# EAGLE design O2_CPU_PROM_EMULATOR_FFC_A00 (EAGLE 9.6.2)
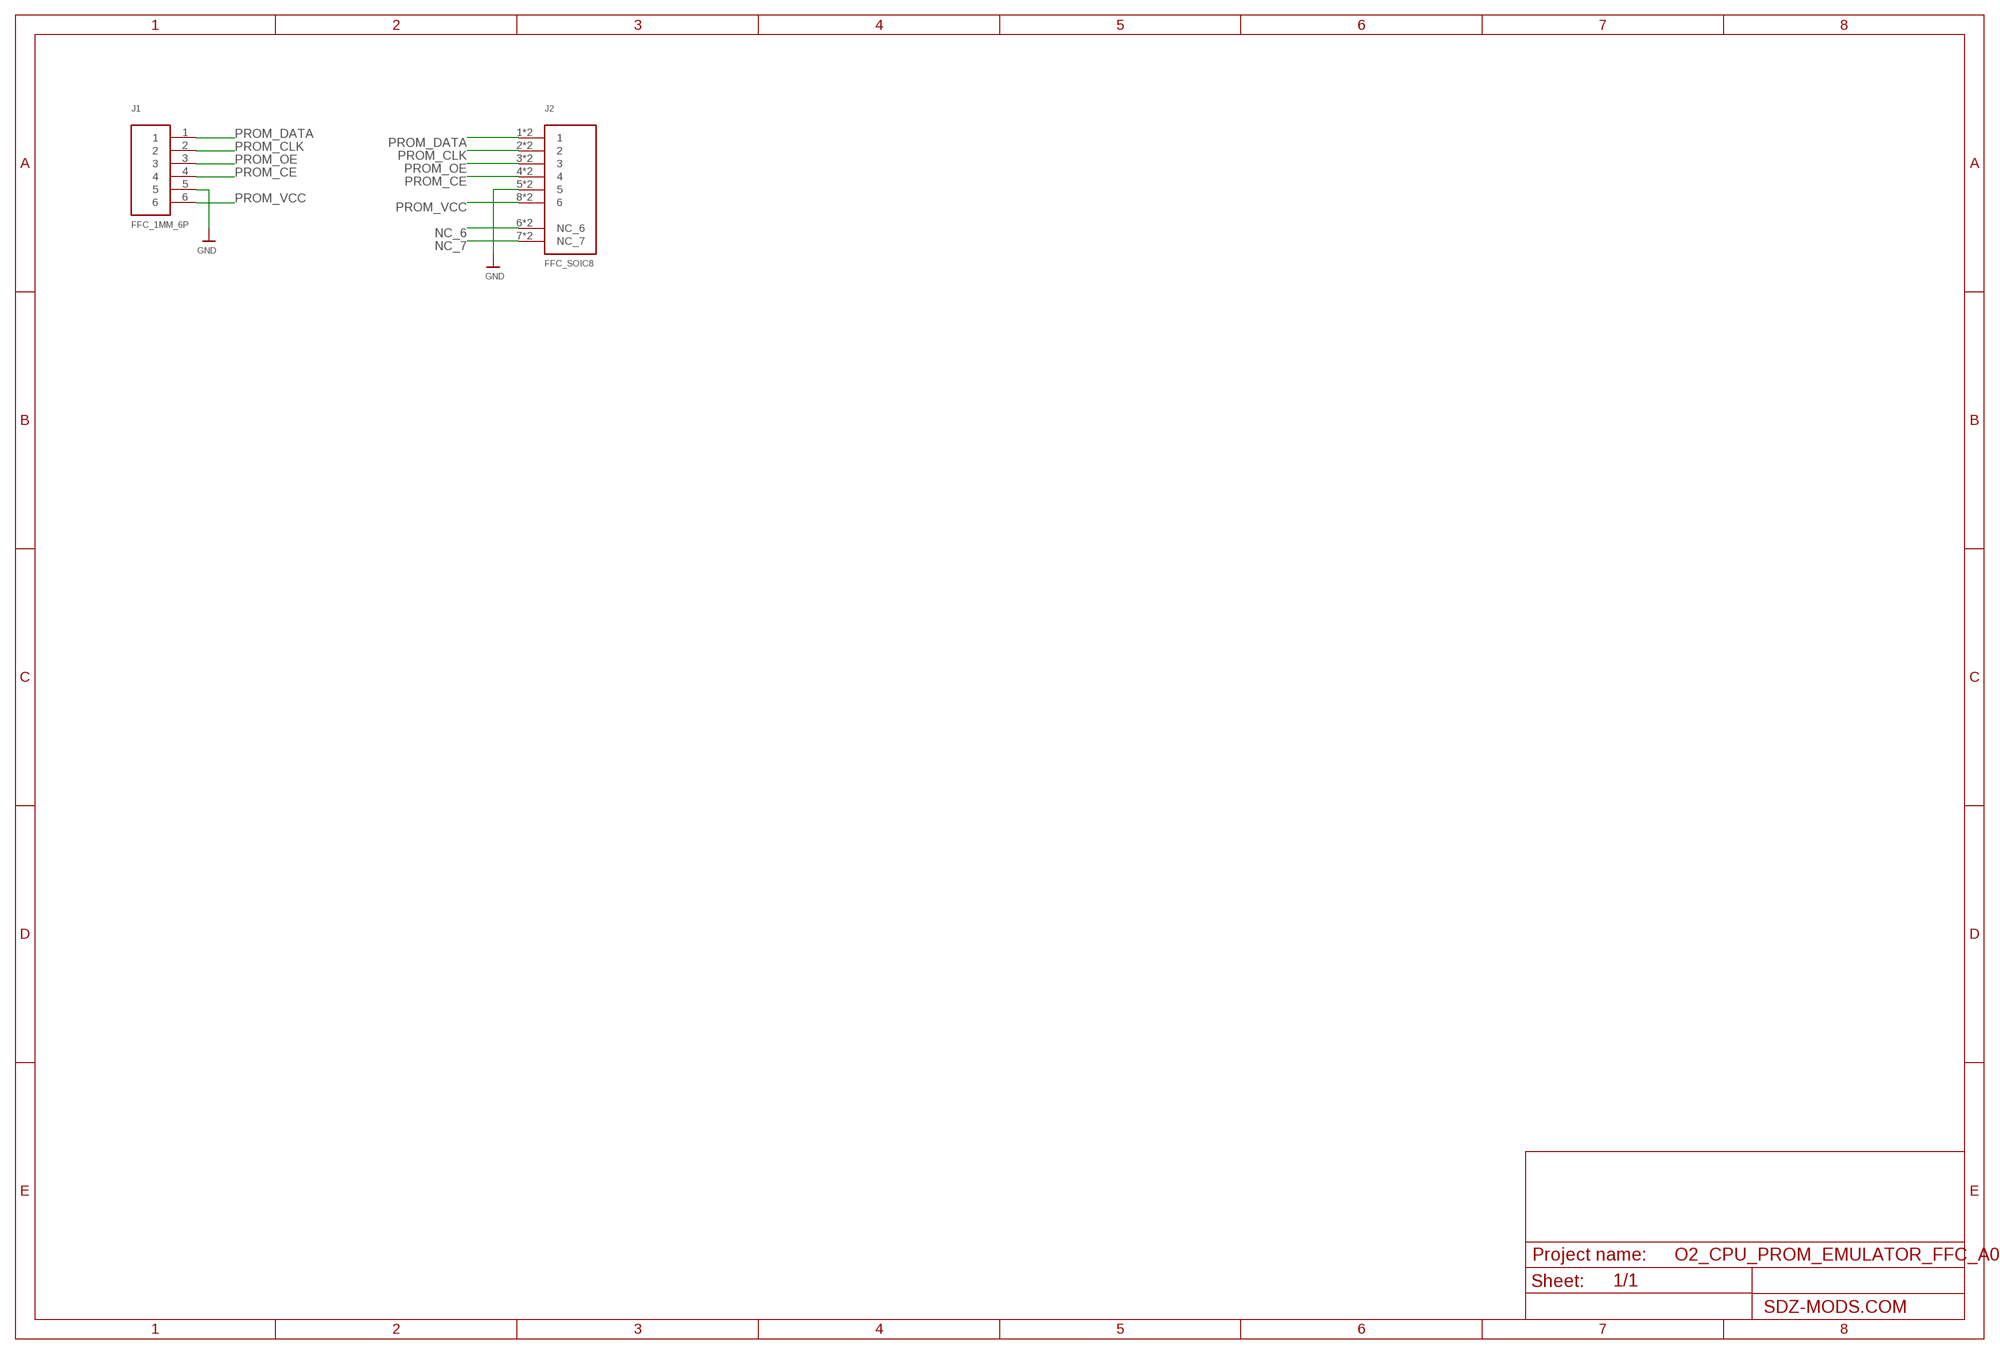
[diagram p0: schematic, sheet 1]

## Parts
J1  FFC_1MM_6P  [FFC_1MM_6P]
J2  FFC_SOIC8  [FFC_SOIC8]

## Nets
GND: J1.5 J2.5 J2.5B
NC_6: J2.6(NC_6) J2.6B(NC_6)
NC_7: J2.7(NC_7) J2.7B(NC_7)
PROM_CE: J1.4 J2.4 J2.4B
PROM_CLK: J1.2 J2.2 J2.2B
PROM_DATA: J1.1 J2.1 J2.1B
PROM_OE: J1.3 J2.3 J2.3B
PROM_VCC: J1.6 J2.8 J2.8B

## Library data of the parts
J1 = FFC_1MM_6P:FFC_1MM_6P
J2 = FFC_SOIC8:FFC_SOIC8

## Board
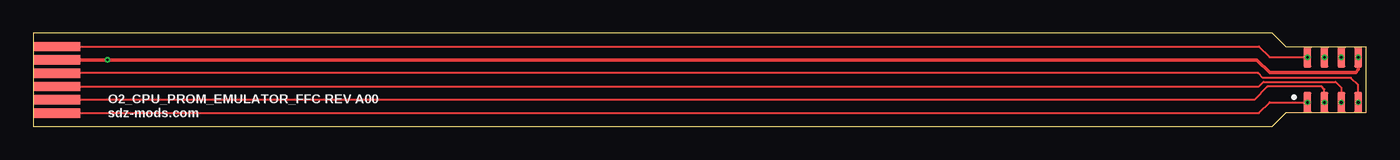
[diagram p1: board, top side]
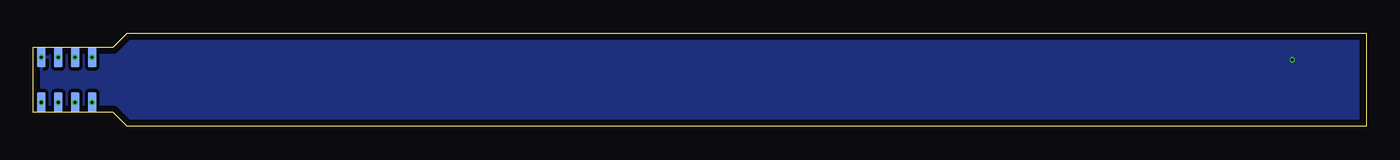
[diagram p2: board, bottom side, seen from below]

Size 100 x 7 mm. Coordinates in mm from the lower left corner, seen from the top.
Outline: 0,0 92.95,0 94,1.05 100,1.05 100,5.95 94,5.95 92.95,7 0,7 0,0
Copper layers (1*16): Top 0.035mm / dielectric 1.5mm / Bottom 0.035mm
Design rules "default *": minimum track width 6mil, minimum drill 0.2mm, track to track 6mil, track to pad 6mil, pad to pad 6mil, via to via 6mil, smd to smd 6mil, copper to edge 20mil, drill to drill 6mil, minimum pad ring 10mil, minimum via ring 0.1mm, stop-mask expansion 4mil, vias tented up to drill 0.35mm, thermal gap 10mil

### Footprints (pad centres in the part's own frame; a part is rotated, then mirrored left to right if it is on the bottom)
FFC_1MM_6P = smd 3.5 x 0.7: 1 0,-2.5; 2 0,-1.5; 3 0,-0.5; 4 0,0.5; 5 0,1.5; 6 0,2.5
FFC_SOIC8 = smd 0.6 x 1.55: 1 -1.905,-1.7; 2 -0.635,-1.7; 3 0.635,-1.7; 4 1.905,-1.7; 5 1.905,1.7; 6 0.635,1.7; 7 -0.635,1.7; 8 -1.905,1.7 | smd 0.6 x 1.55 bottom: 1B -1.905,-1.7; 2B -0.635,-1.7; 3B 0.635,-1.7; 4B 1.905,-1.7; 5B 1.905,1.7; 6B 0.635,1.7; 7B -0.635,1.7; 8B -1.905,1.7

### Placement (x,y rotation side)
J1  1.75,3.5 0 top
J2  97.5,3.5 0 top

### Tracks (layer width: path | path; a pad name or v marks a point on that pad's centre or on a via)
GND  (via drill 0.2)
  Top 0.254: J1.5 v5.55,5 91.8,5 92.75,4.05 99.2,4.05 99.41,4.25 J2.5B
  other vias: 99.41,5.2
  pour Bottom (isolate 0.25): -0.25,7.4 100.5,7.4 100.5,-0.4 -0.25,-0.4
NC_6  (via drill 0.2)
  other vias: 98.14,5.2
NC_7  (via drill 0.2)
  other vias: 96.86,5.2
PROM_CE  (via drill 0.2)
  Top 0.152: J2.4B 99.41,3.1 98.86,3.64 92.26,3.64 91.9,4 J1.4
  other vias: 99.41,1.8
PROM_CLK  (via drill 0.2)
  Top 0.152: J2.2B 96.86,2.79 96.67,2.98 92.58,2.98 91.6,2 J1.2
  other vias: 96.86,1.8
PROM_DATA  (via drill 0.2)
  Top 0.152: J1.1 91.95,1 92.75,1.8 J2.1B
  other vias: 95.59,1.8
PROM_OE  (via drill 0.2)
  Top 0.152: J1.3 91.95,3 92.29,3.34 97.71,3.34 98.14,2.92 J2.3B
  other vias: 98.14,1.8
PROM_VCC  (via drill 0.2)
  Top 0.152: J2.8B 92.75,5.2 91.95,6 J1.6
  other vias: 95.59,5.2

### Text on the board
tPlace: O2_CPU_PROM_EMULATOR_FFC REV A00 / sdz-mods.com
stiffener: 6x7mm stiffener / Stiffener material: polyimide / Stiffener thickness: 0.2mm / Final thickness: 0.29-0.34mm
